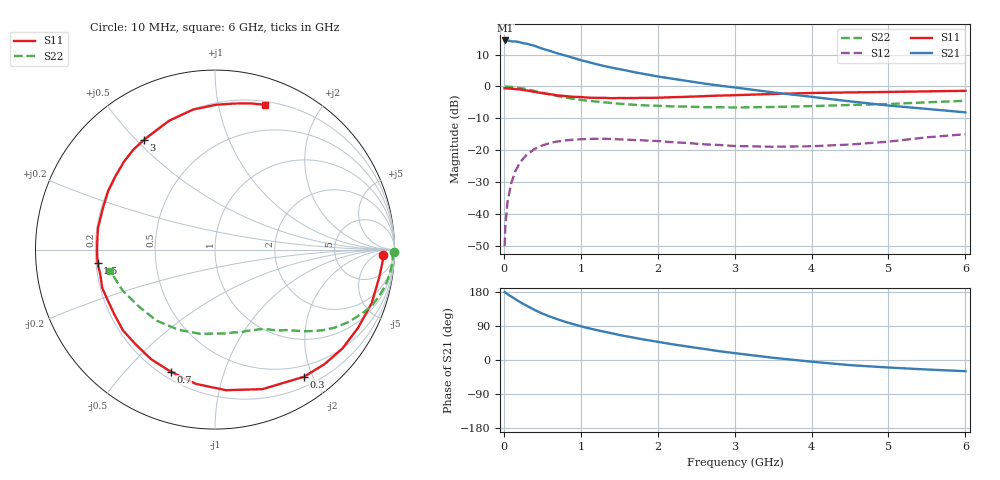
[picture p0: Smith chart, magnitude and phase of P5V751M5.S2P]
! SIEMENS Small Signal Semiconductors
! BFP183
! Si NPN RF Bipolar Junction Transistor in SOT143
! VCE = 0.75 V  IC = 1.5 mA
! Common Emitter S-Parameters:  March  1996
# GHz  S  MA  R  50
!  f  S11  S21  S12  S22
! GHz  MAG  ANG  MAG  ANG  MAG  ANG  MAG  ANG
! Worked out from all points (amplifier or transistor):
!   36 points, 10 MHz to 6 GHz, reference 50 ohm
!   highest |S21| = 14.5 dB at 20 MHz (marker M1)
!   |S21| within 3 dB of that: start of sweep to 559.8 MHz
!   unconditionally stable (mu >= 1): 2.148 GHz to end of sweep
!   at 250 MHz: K = 0.12, MSG = 18.1 dB, |S12| = -22.7 dB
!   at 1.4 GHz: K = 0.64, MSG = 11.2 dB, |S12| = -16.5 dB
!   at 6 GHz: K = 1.20, MAG = 0.7 dB, |S12| = -15.0 dB
!   S11 on the Smith chart (normalised r, x): 10 MHz: 25, -12; 300 MHz: 0.33, -1.87; 700 MHz: 0.24, -0.67; 1.5 GHz: 0.21, -0.05; 3 GHz: 0.20, +0.53; 6 GHz: 0.23, +1.38
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0.01  0.937 -1.8  5.199 179.1  0.0031 85.3  0.9981 -0.8
0.02  0.9368 -3.8  5.282 178.0  0.0065 88.4  0.9897 -1.6
0.05  0.9279 -9.6  5.274 173.4  0.0162 86.4  0.9922 -4.1
0.1  0.9226 -18.9  5.114 167.1  0.0314 78.4  0.9825 -8.1
0.15  0.9084 -28.7  5.095 160.5  0.0468 73.1  0.9688 -12.2
0.2  0.8987 -37.8  4.981 154.2  0.0607 67.7  0.9502 -15.9
0.3  0.8647 -55.0  4.682 143.0  0.0853 58.4  0.9026 -22.5
0.4  0.8213 -71.2  4.348 131.9  0.1044 49.6  0.8487 -28.3
0.5  0.7858 -85.5  3.924 122.6  0.1183 42.1  0.7962 -33.1
0.6  0.7558 -98.0  3.62 114.6  0.1298 35.6  0.7497 -36.8
0.7  0.7236 -109.9  3.299 107.4  0.137 30.3  0.7078 -39.9
0.8  0.7067 -120.3  3.062 100.6  0.1421 25.7  0.6719 -42.6
0.9  0.6885 -129.9  2.823 94.7  0.1459 21.6  0.6401 -44.9
1.1  0.6673 -146.9  2.417 83.8  0.1501 14.8  0.5949 -48.9
1.5  0.6586 -173.7  1.875 66.1  0.1474 5.0  0.5359 -56.0
1.8  0.6631 169.5  1.59 54.7  0.1427 0.8  0.5068 -61.1
2.2  0.6786 151.4  1.319 41.2  0.1332 -3.1  0.486 -68.8
3  0.7288 122.8  0.965 18.1  0.1161 -2.9  0.4679 -87.1
3.5  0.7624 109.5  0.807 5.9  0.1131 1.6  0.4763 -99.7
4.5  0.8068 89.7  0.584 -13.6  0.1225 11.0  0.5126 -129.5
5.5  0.838 76.5  0.444 -25.1  0.159 14.9  0.5634 -156.3
6  0.854 70.9  0.392 -29.5  0.1778 12.4  0.5958 -168.5
